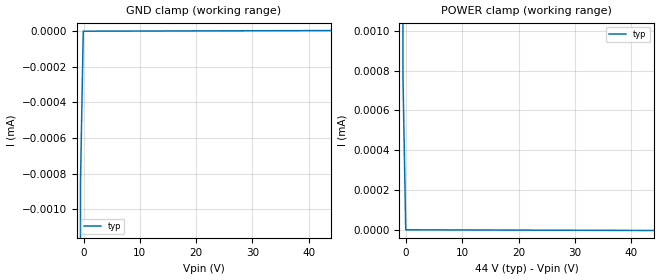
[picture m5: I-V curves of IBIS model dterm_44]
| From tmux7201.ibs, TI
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| dterm_44
[Model]   dterm_44
Model_type   Terminator
|   typ   min   max
C_comp   4.014581e-11   NA   NA
[Voltage Range]   44   NA   NA
[Temperature Range]   27   NA   NA
[Power Clamp Reference]   44   NA   NA
[GND Clamp Reference]   0   NA   NA
[GND Clamp]
|   Voltage   I(typ)   I(min)   I(max)
-5V       -11.65A    NA         NA
-1.04V    -180.6mA   NA         NA
-545.5mV  -861nA     NA         NA
-50.51mV  -1.726nA   NA         NA
44V       1.721nA    NA         NA
[POWER Clamp]
|   Voltage   I(typ)   I(min)   I(max)
-5V       13.27A     NA         NA
-1.04V    178.1mA    NA         NA
-545.5mV  769.7nA    NA         NA
-50.5mV   1.725nA    NA         NA
44V       -1.722nA   NA         NA
